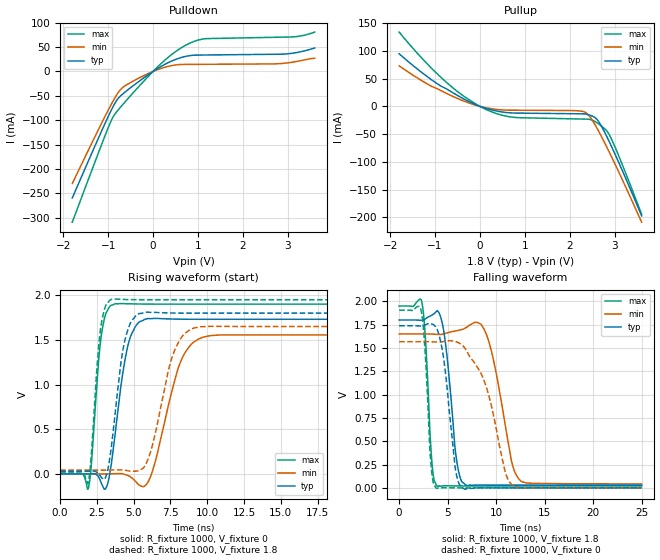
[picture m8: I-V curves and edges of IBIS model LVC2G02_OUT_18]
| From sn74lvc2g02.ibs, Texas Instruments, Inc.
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[Model]   LVC2G02_OUT_18
Model_type  Output
Vref =   0
Rref =   1000
Cref =   30p
Vmeas =   0.9
| variable   typ   min   max
C_comp   9.23pF   6.68pF   16.38pF
| C_pullup   7.81pF   6.68pF   8.36pF
| C_pulldown   10.66pF   6.68pF   16.38pF
[Temperature Range]   40   100   -40
| Ambient temperature   25   85   -40
[Voltage range]   1.8   1.65   1.95
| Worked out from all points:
|   slope of the pulldown table from 0 to 0.27 V, typ, clamps not added: 18.2 ohm
|   slope of the pullup table from 0 to 0.27 V, typ, clamps not added: 41.2 ohm
|   rising waveform, R_fixture 1000, V_fixture 0: 20-80 % time 870ps typ, 1.44ns min, 534ps max; typ from 0 V to 1.73 V
|   falling waveform, R_fixture 1000, V_fixture 1.8: 20-80 % time 915ps typ, 1.64ns min, 553ps max; typ from 1.8 V to 0.029 V
|   rising waveform, R_fixture 1000, V_fixture 1.8: 20-80 % time 794ps typ, 1.32ns min, 506ps max; typ from 0.029 V to 1.8 V
|   falling waveform, R_fixture 1000, V_fixture 0: 20-80 % time 1.06ns typ, 2.32ns min, 550ps max; typ from 1.74 V to 0 V
[Pulldown]
| LVC2G02_OUT_18
|   Voltage   I(typ)   I(min)   I(max)
-1.8V     -259.1mA   -229.6mA   -308.8mA
-975mV    -87.66mA   -75.04mA   -109.8mA
-875mV    -69.28mA   -58.05mA   -90.65mA
-735mV    -50.98mA   -38.25mA   -74.26mA
-595mV    -40.11mA   -27.77mA   -59.37mA
-185mV    -11.71mA   -7.652mA   -17.82mA
405mV     20.9mA     11.73mA    33.97mA
775mV     31.75mA    14.39mA    55.98mA
1.11V     33.57mA    14.57mA    66.34mA
2.935V    35.63mA    16.87mA    70.3mA
3.265V    39.89mA    21.62mA    72.33mA
3.6V      48.06mA    27.06mA    80.56mA
[Pullup]
| LVC2G02_OUT_18
|   Voltage   I(typ)   I(min)   I(max)
-1.8V     95.04mA    73.2mA     134.2mA
-1.265V   59.33mA    44.93mA    84.52mA
-775mV    32.87mA    24.71mA    45.48mA
-350mV    13.07mA    9.365mA    17.89mA
125mV     -3.364mA   -2.274mA   -5.1mA
765mV     -11.99mA   -6.831mA   -19.76mA
2.085V    -13.21mA   -7.553mA   -22.48mA
2.36V     -13.9mA    -11.34mA   -22.95mA
2.605V    -23.44mA   -39.14mA   -29.49mA
2.865V    -61.25mA   -80.13mA   -49.02mA
3.115V    -105.7mA   -122.6mA   -94.24mA
3.6V      -197.4mA   -209mA     -194.8mA
[Ramp]
| LVC2G02_OUT_18
| variable   typ   min   max
dV/dt_r   1.15/9.48E-10   1.02/1.59E-09   1.24/5.98E-10
dV/dt_f   1.12/1.05E-09   1.04/1.83E-09   1.20/6.21E-10
R_load = 1000
[Rising Waveform]
| LVC2G02_OUT_18
R_fixture =   1000
C_fixture =   0
L_fixture =   0
V_fixture =   0
V_fixture_min = 0
V_fixture_max = 0
|   Time   V(typ)   V(min)   V(max)
0s        -89.54nV   -611.6nV   20.87nV
1.92ns    638.6uV    -59.22uV   -158.3mV
2.765ns   -88.96mV   -177.8uV   1.511V
3.48ns    113.4mV    1.609mV    1.889V
4.525ns   1.378V     -12.58mV   1.905V
5.45ns    1.708V     -131.6mV   1.902V
6.26ns    1.74V      23.66mV    1.901V
8.17ns    1.732V     1.249V     1.901V
9.45ns    1.731V     1.514V     1.901V
24.99ns   1.731V     1.556V     1.901V
[Falling Waveform]
| LVC2G02_OUT_18
R_fixture =   1000
C_fixture =   0
L_fixture =   0
V_fixture =   1.8
V_fixture_min = 1.65
V_fixture_max = 1.95
|   Time   V(typ)   V(min)   V(max)
0s        1.8V       1.65V      1.95V
2.34ns    1.797V     1.65V      1.992V
3.385ns   1.853V     1.649V     264.4mV
3.92ns    1.901V     1.646V     17.42mV
4.665ns   1.637V     1.653V     22.27mV
5.795ns   397.2mV    1.682V     20.87mV
6.53ns    57.58mV    1.7V       20.44mV
9.015ns   30.44mV    1.64V      20.47mV
12.5ns    29.26mV    76.82mV    20.47mV
24.99ns   29.16mV    42.62mV    20.47mV
[Rising Waveform]
| LVC2G02_OUT_18
R_fixture =   1000
C_fixture =   0
L_fixture =   0
V_fixture =   1.8
V_fixture_min = 1.65
V_fixture_max = 1.95
|   Time   V(typ)   V(min)   V(max)
0s        29.14mV    42.51mV    20.46mV
1.905ns   29.66mV    42.46mV    -95.2mV
2.725ns   -20.99mV   42.4mV     1.596V
3.445ns   258.5mV    43.9mV     1.951V
4.34ns    1.452V     42.12mV    1.954V
5.33ns    1.792V     35.24mV    1.951V
6.16ns    1.808V     255.8mV    1.95V
7.715ns   1.801V     1.355V     1.95V
8.91ns    1.8V       1.622V     1.95V
24.99ns   1.8V       1.65V      1.95V
[Falling Waveform]
| LVC2G02_OUT_18
R_fixture =   1000
C_fixture =   0
L_fixture =   0
V_fixture =   0
V_fixture_min = 0
V_fixture_max = 0
|   Time   V(typ)   V(min)   V(max)
0s        1.738V     1.567V     1.905V
2.275ns   1.736V     1.567V     1.898V
3.28ns    1.759V     1.566V     251.4mV
3.845ns   1.713V     1.565V     -4.261mV
4.625ns   1.359V     1.57V      1.012mV
5.805ns   198.5mV    1.569V     65.89uV
6.625ns   -6.312mV   1.518V     -80.39uV
8.835ns   385.9uV    1.126V     4.098uV
11.76ns   51.06uV    19.91mV    7.306uV
24.99ns   16.67uV    49.65uV    6.055uV
